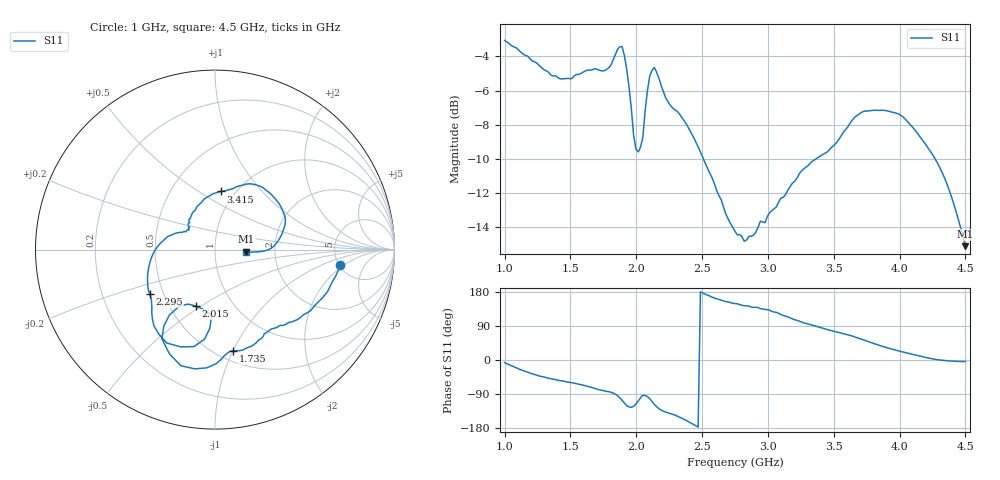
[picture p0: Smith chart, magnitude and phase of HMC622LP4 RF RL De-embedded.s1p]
! Hittite Microwave Corporation
! 20 Alpha Road
! Chelmsford, MA 01824
! http://www.hittite.com
! Tel: 978-250-3343
! Fax: 978-250-3373
! Device:  HMC622LP4
! Description:  GaAS MMIC MIXER With integrated IF/LO Amplifier
! Frequency:  1.8-  3.9 GHz
! Package:
! Data:  The device was measured on evaluation board 119242
!  The evaluation circuit board was modeled and simulated.  This was use
!  to removed the evaluation board circuit from the measured data.
!  The reference plane is the center of the package pin.
! Misc:
! Date Measured:  06-09-2009
! Date:  08-24-2009
! Note:
!  Hittite supplies this data as a sample of measured data at the package pin for
!  for this package product.  Your particular data for this product may vary.
!  Data was taken at 25 degrees C.
!  Hittite reserves the right to change this data at anytime.
# MHz S MA R 50
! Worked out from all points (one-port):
!   201 points, 1 GHz to 4.5 GHz, reference 50 ohm
!   lowest |S11| = -15.1 dB at 4.5 GHz (marker M1), VSWR 1.43, Z = 71.2 - j1.82 ohm
!   |S11| at or under -10 dB: 2.51 GHz to 3.365 GHz (855.1 MHz wide, 29.1 % of centre); 4.27 GHz to end of sweep
!   S11 on the Smith chart (normalised r, x): 1 GHz: 5.14, -1.72; 1.735 GHz: 0.60, -1.00; 2.015 GHz: 0.67, -0.48; 2.295 GHz: 0.42, -0.26; 3.415 GHz: 0.86, +0.62; 4.5 GHz: 1.42, -0.04
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1000  0.7028 -6.9
1175  0.6322 -32.5
1437.5  0.5426 -55.1
1595  0.5673 -66.0
1735  0.573 -79.7
1822.5  0.6139 -86.9
1875  0.6741 -99.7
1892.5  0.6741 -106.4
1927.5  0.5786 -120.8
1980  0.3704 -122.2
2015  0.3316 -108.5
2050  0.366 -92.9
2067.5  0.4391 -93.8
2102.5  0.5528 -102.2
2120  0.5746 -109.4
2172.5  0.5444 -128.7
2295  0.4398 -145.5
2312.5  0.4355 -148.2
2522.5  0.3079 173.8
2750  0.1942 149.0
2890  0.189 138.5
3187.5  0.2688 108.2
3415  0.3256 84.0
3625  0.4028 64.8
3870  0.4393 36.0
4062.5  0.4061 17.9
4325  0.2877 -0.8
4500  0.1757 -4.0
